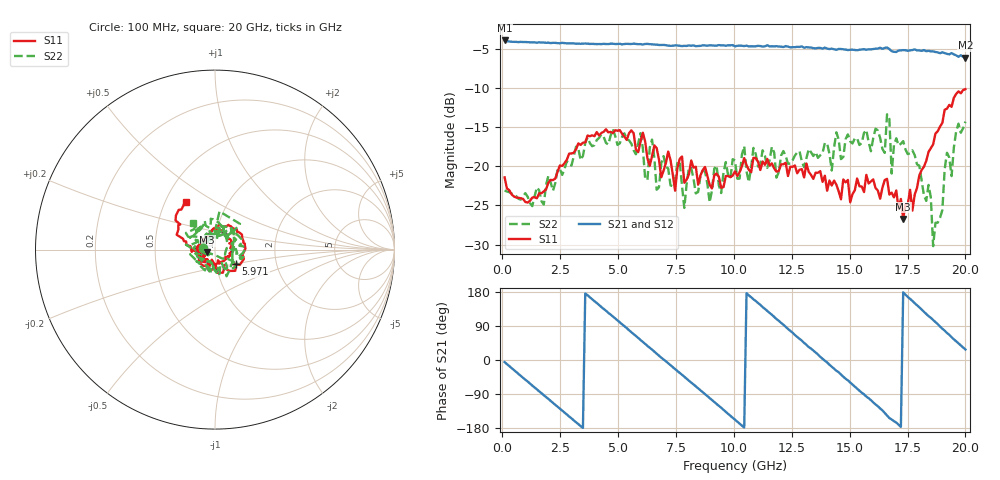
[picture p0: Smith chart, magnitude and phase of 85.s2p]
!Agilent Technologies,N5230C,MY49001569,A.09.33.09
!Agilent N5230C: A.09.33.09
!Date: Monday, July 20, 2015 19:52:49
!Correction: S11(Full 2 Port(1,2))
!S21(Full 2 Port(1,2))
!S12(Full 2 Port(1,2))
!S22(Full 2 Port(1,2))
!S2P File: Measurements: S11, S21, S12, S22:
# Hz S  dB  R 50
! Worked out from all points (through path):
!   201 points, 100 MHz to 20 GHz, reference 50 ohm
!   highest |S21| = -3.97 dB at 100 MHz (marker M1); lowest = -6.2 dB at 20 GHz (marker M2)
!   group delay of S21, straight-line fit = 145 ps
!   lowest |S11| = -26.7 dB at 17.31 GHz (marker M3), VSWR 1.10, Z = 45.8 - j1.48 ohm
!   |S11| at or under -10 dB: start of sweep to end of sweep
!   |S22| runs from -30.2 to -13.4 dB; largest |S21 - S12| = 0.018
!   S11 on the Smith chart (normalised r, x): 100 MHz: 0.84, +0.02; 5.971 GHz: 1.25, -0.21; 20 GHz: 0.64, +0.37
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1e8  -21.42 172.6  -3.97 -5.6  -3.99 -5.6  -23.08 171.6
1.7915e9  -23.21 124.4  -4.23 -92.7  -4.27 -92.8  -24.89 115.7
3.483e9  -17.01 66.6  -4.37 -179.2  -4.36 -179.4  -18.69 60.3
4.7765e9  -15.78 13.4  -4.39 114.8  -4.41 114.6  -15.30 1.9
5.9705e9  -16.86 -34.9  -4.44 52.8  -4.44 53.2  -15.79 -66.5
6.1695e9  -16.84 -55.8  -4.42 42.6  -4.41 42.7  -21.54 -63.4
6.468e9  -18.70 -63.9  -4.46 27.4  -4.50 27.3  -16.61 -81.6
6.7665e9  -19.16 -86.2  -4.55 11.4  -4.53 11.6  -22.69 -107.0
8.657e9  -20.50 -157.4  -4.59 -85.0  -4.59 -84.7  -20.56 149.3
8.9555e9  -22.37 170.8  -4.59 -100.3  -4.62 -100.2  -24.62 132.9
1.005e10  -20.67 110.3  -4.72 -157.6  -4.64 -157.2  -19.27 71.4
1.1841e10  -20.69 38.3  -4.70 108.0  -4.72 108.5  -21.46 -36.6
1.3433e10  -21.62 -15.8  -4.95 25.0  -4.93 25.0  -18.70 -143.0
1.5224e10  -23.07 -99.3  -5.18 -70.1  -5.21 -69.0  -16.45 121.7
1.65175e10  -21.76 -155.7  -4.92 -139.5  -4.82 -138.8  -18.31 88.1
1.67165e10  -23.61 -154.1  -5.07 -153.3  -5.06 -152.6  -13.98 45.8
1.6816e10  -23.37 -147.1  -5.34 -156.9  -5.35 -156.8  -20.93 41.6
1.73135e10  -26.72 -159.5  -5.21 178.4  -5.25 178.2  -16.80 45.5
1.8408e10  -18.18 -178.7  -5.29 115.7  -5.29 117.6  -22.39 -42.1
1.8607e10  -17.21 172.3  -5.36 105.6  -5.31 105.7  -30.20 -87.8
1.9204e10  -12.66 151.2  -5.68 71.4  -5.58 72.3  -18.29 176.5
2e10  -10.18 121.7  -6.16 27.7  -6.07 28.0  -14.32 129.7
